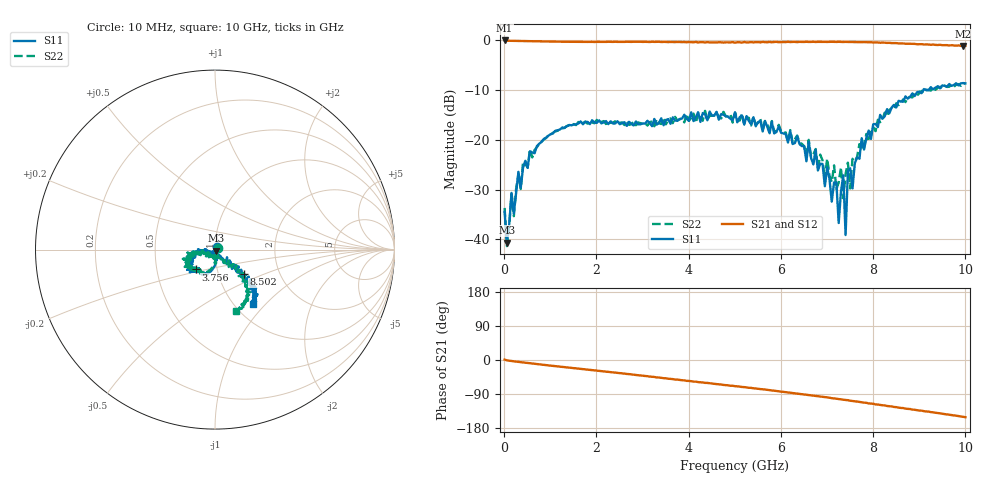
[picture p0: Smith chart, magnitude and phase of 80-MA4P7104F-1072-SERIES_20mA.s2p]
!Agilent Technologies,E8364C,MY48140145,A.09.42.15
!Agilent E8364C: A.09.42.15
!Date: Wednesday, December 02, 2020 07:34:42
!Correction: S11(Full 2 Port(1,2))
!S21(Full 2 Port(1,2))
!S12(Full 2 Port(1,2))
!S22(Full 2 Port(1,2))
!S2P File: Measurements: S11, S21, S12, S22:
# Hz S  dB  R 50
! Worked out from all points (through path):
!   201 points, 10 MHz to 10 GHz, reference 50 ohm
!   highest |S21| = -0.10 dB at 10 MHz (marker M1); lowest = -1.2 dB at 9.95 GHz (marker M2)
!   group delay of S21, straight-line fit = 41 ps
!   lowest |S11| = -40.6 dB at 59.95 MHz (marker M3), VSWR 1.02, Z = 50.7 - j0.587 ohm
!   |S11| at or under -10 dB: start of sweep to 9.092 GHz; 9.136 GHz to 9.207 GHz (70.87 MHz wide, 0.773 % of centre)
!   |S22| runs from -41.4 to -8.6 dB; largest |S21 - S12| = 0.023
!   S11 on the Smith chart (normalised r, x): 10 MHz: 1.02, +0.03; 3.756 GHz: 0.79, -0.18; 8.502 GHz: 1.32, -0.38; 10 GHz: 1.21, -0.84
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1e7  -34.47 49.5  -0.10 1.1  -0.15 -0.2  -33.70 34.4
5.995e7  -40.64 -38.5  -0.15 -1.0  -0.14 -1.0  -41.37 -40.9
1.5985e8  -30.69 -67.9  -0.17 -2.8  -0.16 -2.7  -30.88 -67.2
2.098e8  -34.84 -55.9  -0.18 -3.5  -0.17 -3.5  -35.36 -65.0
3.097e8  -26.45 -79.9  -0.21 -5.0  -0.21 -5.0  -26.89 -77.2
5.5945e8  -22.35 -89.1  -0.25 -8.6  -0.24 -8.6  -21.91 -88.6
1.7083e9  -16.91 -113.2  -0.38 -24.1  -0.36 -23.9  -16.67 -118.6
3.35665e9  -16.65 -133.4  -0.36 -46.2  -0.38 -46.5  -16.72 -127.2
3.75625e9  -16.22 -134.4  -0.39 -51.8  -0.43 -52.0  -16.16 -131.8
5.005e9  -14.51 -151.0  -0.55 -69.1  -0.50 -68.9  -14.58 -164.0
6.7033e9  -24.96 -174.8  -0.37 -94.2  -0.34 -93.9  -23.00 -177.8
7.2028e9  -28.59 -93.8  -0.39 -102.0  -0.36 -101.9  -29.96 -98.7
7.25275e9  -36.72 -143.1  -0.37 -103.1  -0.36 -102.9  -28.59 -144.2
7.35265e9  -27.16 -65.7  -0.40 -104.8  -0.37 -104.4  -31.75 -73.0
7.4026e9  -39.14 -92.7  -0.39 -105.5  -0.38 -105.6  -26.92 -104.5
7.45255e9  -26.32 -75.1  -0.40 -106.0  -0.39 -106.4  -24.62 -66.0
7.5025e9  -25.74 -50.1  -0.41 -107.5  -0.37 -107.0  -29.80 -61.1
7.7023e9  -23.83 -52.0  -0.42 -110.5  -0.44 -110.8  -20.89 -55.0
8.35165e9  -14.72 -37.5  -0.57 -122.0  -0.60 -122.0  -14.04 -48.2
8.5015e9  -13.55 -40.7  -0.63 -124.4  -0.66 -124.8  -12.70 -46.7
9.95005e9  -8.64 -52.3  -1.19 -150.1  -1.22 -149.9  -8.62 -71.1
1e10  -8.70 -55.1  -1.18 -150.9  -1.18 -150.9  -8.80 -70.8
